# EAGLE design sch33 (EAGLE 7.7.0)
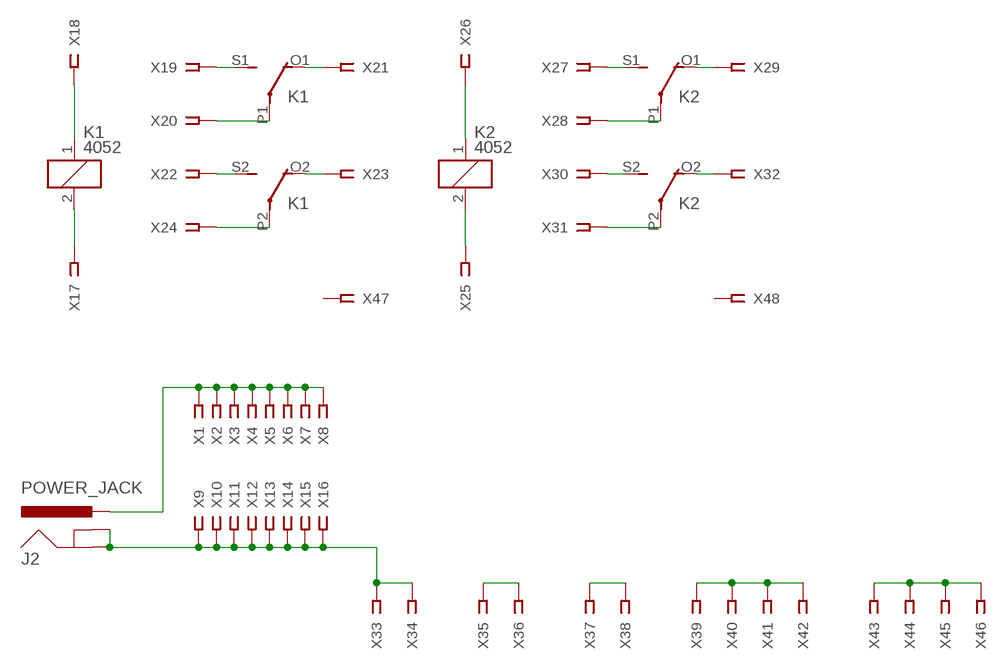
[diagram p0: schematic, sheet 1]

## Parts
J2  POWER_JACK  [POWER_JACK_PTH]
K1  4052  [F4052]
K2  4052  [F4052]
X1  SSW-101-02-S-S  [SSW-101-02-S-S]
X2  SSW-101-02-S-S  [SSW-101-02-S-S]
X3  SSW-101-02-S-S  [SSW-101-02-S-S]
X4  SSW-101-02-S-S  [SSW-101-02-S-S]
X5  SSW-101-02-S-S  [SSW-101-02-S-S]
X6  SSW-101-02-S-S  [SSW-101-02-S-S]
X7  SSW-101-02-S-S  [SSW-101-02-S-S]
X8  SSW-101-02-S-S  [SSW-101-02-S-S]
X9  SSW-101-02-S-S  [SSW-101-02-S-S]
X10  SSW-101-02-S-S  [SSW-101-02-S-S]
X11  SSW-101-02-S-S  [SSW-101-02-S-S]
X12  SSW-101-02-S-S  [SSW-101-02-S-S]
X13  SSW-101-02-S-S  [SSW-101-02-S-S]
X14  SSW-101-02-S-S  [SSW-101-02-S-S]
X15  SSW-101-02-S-S  [SSW-101-02-S-S]
X16  SSW-101-02-S-S  [SSW-101-02-S-S]
X17  SSW-101-02-S-S  [SSW-101-02-S-S]
X18  SSW-101-02-S-S  [SSW-101-02-S-S]
X19  SSW-101-02-S-S  [SSW-101-02-S-S]
X20  SSW-101-02-S-S  [SSW-101-02-S-S]
X21  SSW-101-02-S-S  [SSW-101-02-S-S]
X22  SSW-101-02-S-S  [SSW-101-02-S-S]
X23  SSW-101-02-S-S  [SSW-101-02-S-S]
X24  SSW-101-02-S-S  [SSW-101-02-S-S]
X25  SSW-101-02-S-S  [SSW-101-02-S-S]
X26  SSW-101-02-S-S  [SSW-101-02-S-S]
X27  SSW-101-02-S-S  [SSW-101-02-S-S]
X28  SSW-101-02-S-S  [SSW-101-02-S-S]
X29  SSW-101-02-S-S  [SSW-101-02-S-S]
X30  SSW-101-02-S-S  [SSW-101-02-S-S]
X31  SSW-101-02-S-S  [SSW-101-02-S-S]
X32  SSW-101-02-S-S  [SSW-101-02-S-S]
X33  SSW-101-02-S-S  [SSW-101-02-S-S]
X34  SSW-101-02-S-S  [SSW-101-02-S-S]
X35  SSW-101-02-S-S  [SSW-101-02-S-S]
X36  SSW-101-02-S-S  [SSW-101-02-S-S]
X37  SSW-101-02-S-S  [SSW-101-02-S-S]
X38  SSW-101-02-S-S  [SSW-101-02-S-S]
X39  SSW-101-02-S-S  [SSW-101-02-S-S]
X40  SSW-101-02-S-S  [SSW-101-02-S-S]
X41  SSW-101-02-S-S  [SSW-101-02-S-S]
X42  SSW-101-02-S-S  [SSW-101-02-S-S]
X43  SSW-101-02-S-S  [SSW-101-02-S-S]
X44  SSW-101-02-S-S  [SSW-101-02-S-S]
X45  SSW-101-02-S-S  [SSW-101-02-S-S]
X46  SSW-101-02-S-S  [SSW-101-02-S-S]
X47  SSW-101-02-S-S  [SSW-101-02-S-S]
X48  SSW-101-02-S-S  [SSW-101-02-S-S]

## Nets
N$1 [power]: J2.PWR X1.1 X2.1 X3.1 X4.1 X5.1 X6.1 X7.1 X8.1
N$2 [power]: J2.GND J2.GNDBREAK X9.1 X10.1 X11.1 X12.1 X13.1 X14.1 X15.1 X16.1 X33.1 X34.1
N$3: K1.1 X18.1
N$4: K1.2 X17.1
N$5: K1.S1(2:S) X19.1
N$6: K1.P1(2:P) X20.1
N$7: K1.O1(2:O) X21.1
N$8: K1.S2(3:S) X22.1
N$9: K1.P2(3:P) X24.1
N$10: K1.O2(3:O) X23.1
N$11: K2.2 X25.1
N$12: K2.1 X26.1
N$13: K2.S1(2:S) X27.1
N$14: K2.P1(2:P) X28.1
N$15: K2.O1(2:O) X29.1
N$16: K2.S2(3:S) X30.1
N$17: K2.P2(3:P) X31.1
N$18: K2.O2(3:O) X32.1
N$19: X35.1 X36.1
N$20: X37.1 X38.1
N$21: X39.1 X40.1 X41.1 X42.1
N$22: X43.1 X44.1 X45.1 X46.1
Unconnected: X47.1 X48.1

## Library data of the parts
J2 = SparkFun-Connectors:POWER_JACK: Power Jack Connector This is the standard 5.5mm barrel jack for power. The PTH is the most common, proven, reliable, footprint. The Slot footprint only works if the mill layer is transmitted to the PCB fab house so be warned. Here are the connectors we sell at SparkFun: DC Barrel Power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; PROD_ID: CONN-08197
K1 K2 = relay:4052: RELAY 2 x switch, Finder; OC_FARNELL: unknown; OC_NEWARK: unknown
X1-X48 = con-samtec:SSW-101-02-S-S: THROUGH-HOLE .025" SQ POST SOCKET; MPN: SSW-101-02-S-S; OC_FARNELL: unknown; OC_NEWARK: 11P9336

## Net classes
0 default: width 1 mm, clearance 1.5 mm
1 power: width 1 mm, clearance 1.5 mm

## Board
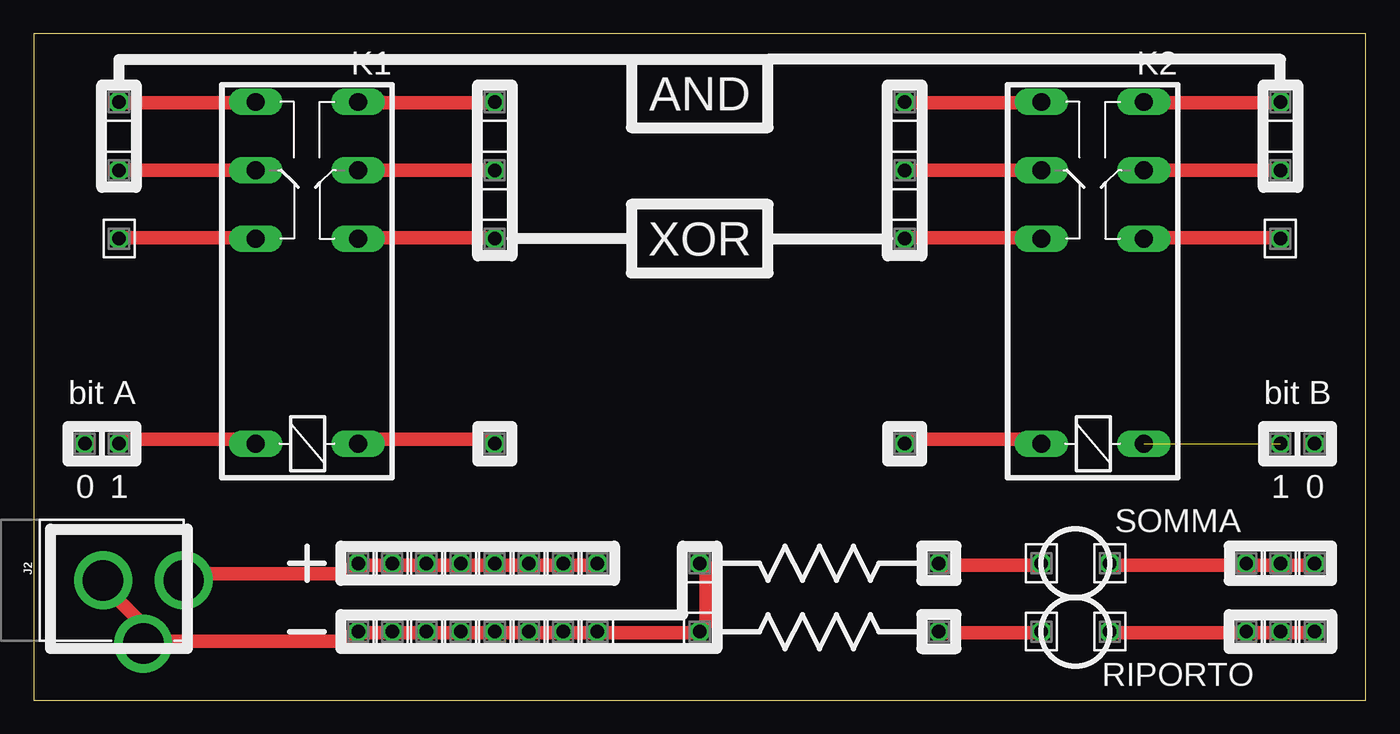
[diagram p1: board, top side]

Size 99.06 x 49.53 mm. Coordinates in mm from the lower left corner, seen from the top.
Outline: 0,0 99.04,0 99.06,49.53 0,49.53 0,0
Copper layers (1*16): Top 0.035mm / dielectric 1.5mm / Bottom 0.035mm
Design rules "default": minimum track width 10mil, minimum drill 24mil, track to track 8mil, track to pad 8mil, pad to pad 8mil, via to via 8mil, smd to smd 8mil, copper to edge 40mil, drill to drill 8mil, minimum pad ring 10mil, minimum via ring 8mil, stop-mask expansion 4mil, vias tented up to drill 0mil, thermal gap 10mil

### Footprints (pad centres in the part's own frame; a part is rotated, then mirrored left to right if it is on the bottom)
POWER_JACK_PTH = drill 2.997 pad 4.318: GND 0,7.7; GNDBREAK 4.7,10.7; PWR 0,13.7
F4052 = drill 1.321 long: 1 -3.81,3.81; 2 -3.81,-3.81; O1 11.43,-3.81; O2 11.43,3.81; P1 16.51,-3.81; P2 16.51,3.81; S1 21.59,-3.81; S2 21.59,3.81
SSW-101-02-S-S = drill 1 pad 1.5 octagon: 1 0,0

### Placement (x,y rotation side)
J2  -2.54,8.89 270 top
K1  20.32,22.86 90 top
K2  78.74,22.86 90 top
X1  24.13,10.16 90 top
X2  26.67,10.16 90 top
X3  29.21,10.16 90 top
X4  31.75,10.16 90 top
X5  34.29,10.16 90 top
X6  36.83,10.16 90 top
X7  39.37,10.16 90 top
X8  41.91,10.16 90 top
X9  24.13,5.08 270 top
X10  26.67,5.08 270 top
X11  29.21,5.08 270 top
X12  31.75,5.08 270 top
X13  34.29,5.08 270 top
X14  36.83,5.08 270 top
X15  39.37,5.08 270 top
X16  41.91,5.08 270 top
X17  34.29,19.05 90 top
X18  6.35,19.05 90 top
X19  34.29,44.45 90 top
X20  34.29,39.37 90 top
X21  34.29,34.29 90 top
X22  6.35,44.45 90 top
X23  6.35,34.29 90 top
X24  6.35,39.37 90 top
X25  92.71,19.05 90 top
X26  64.77,19.05 90 top
X27  92.71,44.45 90 top
X28  92.71,39.37 90 top
X29  92.71,34.29 90 top
X30  64.77,44.45 90 top
X31  64.77,39.37 90 top
X32  64.77,34.29 90 top
X33  49.53,5.08 270 top
X34  49.53,10.16 270 top
X35  67.31,5.08 270 top
X36  74.93,5.08 270 top
X37  67.31,10.16 270 top
X38  74.93,10.16 270 top
X39  80.01,5.08 270 top
X40  92.71,5.08 270 top
X41  95.25,5.08 270 top
X42  90.17,5.08 90 top
X43  80.01,10.16 270 top
X44  90.17,10.16 270 top
X45  92.71,10.16 270 top
X46  95.25,10.16 270 top
X47  3.81,19.05 90 top
X48  95.25,19.05 90 top

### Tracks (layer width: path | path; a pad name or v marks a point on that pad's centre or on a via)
N$1
  Top 1: X8.1 41.88,10 39.38,10 X7.1 38.75,10 36.88,10 X6.1 36.25,10 34.38,10 X5.1 33.75,10 31.88,10 X4.1 31.25,10 29.38,10 X3.1 28.75,10 26.88,10 X2.1 26.25,10 24.38,10 X1.1 23.75,10 23.12,9.38 11.25,9.38 J2.PWR
N$2
  Top 1: J2.GND 5,8.75 8.12,5.62 8.12,4.38 J2.GNDBREAK 8.75,4.38 23.12,4.38 23.75,5 X9.1 24.38,5 26.25,5 X10.1 26.88,5 28.75,5 X11.1 29.38,5 31.25,5 X12.1 31.88,5 33.75,5 X13.1 34.38,5 36.25,5 X14.1 36.88,5 38.75,5 X15.1 39.38,5 41.88,5 X16.1 42.5,5 49.38,5 X33.1 50,5.62 50,10 X34.1
N$3
  Top 1: X18.1 6.88,19.38 16.25,19.38 K1.1
N$4
  Top 1: X17.1 33.75,19.38 24.38,19.38 K1.2
N$5
  Top 1: X19.1 33.75,44.38 24.38,44.38 K1.S1
N$6
  Top 1: X20.1 33.75,39.38 24.38,39.38 K1.P1
N$7
  Top 1: X21.1 33.75,34.38 24.38,34.38 K1.O1
N$8
  Top 1: X22.1 6.88,44.38 16.25,44.38 K1.S2
N$9
  Top 1: X24.1 6.88,39.38 16.25,39.38 K1.P2
N$10
  Top 1: X23.1 6.88,34.38 16.25,34.38 K1.O2
N$11  (1 unrouted)
N$12
  Top 1: X26.1 65,19.38 74.38,19.38 K2.1
N$13
  Top 1: X27.1 92.5,44.38 83.12,44.38 K2.S1
N$14
  Top 1: X28.1 92.5,39.38 83.12,39.38 K2.P1
N$15
  Top 1: X29.1 92.5,34.38 83.12,34.38 K2.O1
N$16
  Top 1: X30.1 65,44.38 74.38,44.38 K2.S2
N$17
  Top 1: X31.1 65,39.38 74.38,39.38 K2.P2
N$18
  Top 1: X32.1 65,34.38 74.38,34.38 K2.O2
N$19
  Top 1: X35.1 67.5,5 74.38,5 X36.1
N$20
  Top 1: X37.1 67.5,10 74.38,10 X38.1
N$21
  Top 1: X41.1 95,5 93.12,5 X40.1 92.5,5 90.62,5 X42.1 90,5 80.62,5 X39.1
N$22
  Top 1: X46.1 95,10 93.12,10 X45.1 92.5,10 90.62,10 X44.1 90,10 80.62,10 X43.1

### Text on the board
tNames: AND | XOR | bit A | bit B | 0 | 1 | 1 | 0 | SOMMA | RIPORTO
